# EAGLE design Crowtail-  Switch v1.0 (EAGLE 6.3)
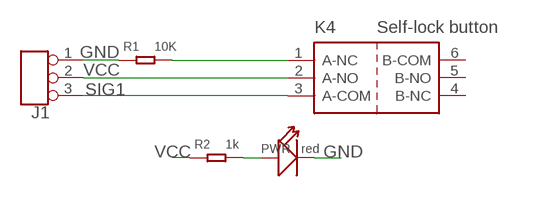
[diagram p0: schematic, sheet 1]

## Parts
J1  TINKER_3P_DIP  [3P_2.0_DIP]
K4  Self-lock button  BUTTON-6P  [6P-2CH-8X8]
PWR  red  LED'0603'  [LED-0603]
R1  10K  R-0603  [0603]
R2  1k  R-0603  [0603]

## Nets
GND: J1.1 PWR.- R1.1
N$1: PWR.+ R2.2
N$2: K4.1(A-NC) R1.2
SIG1: J1.3 K4.3(A-COM)
VCC: J1.2 K4.2(A-NO) R2.1
Unconnected: K4.4(B-NC) K4.5(B-NO) K4.6(B-COM)

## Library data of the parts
J1 = Connector:TINKER_3P_DIP
K4 = Discrete:BUTTON-6P
PWR = Discrete:LED*
R1 R2 = Discrete:R*

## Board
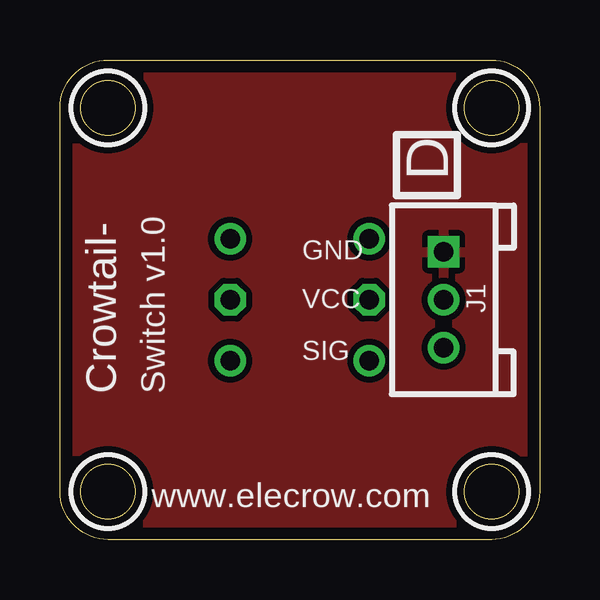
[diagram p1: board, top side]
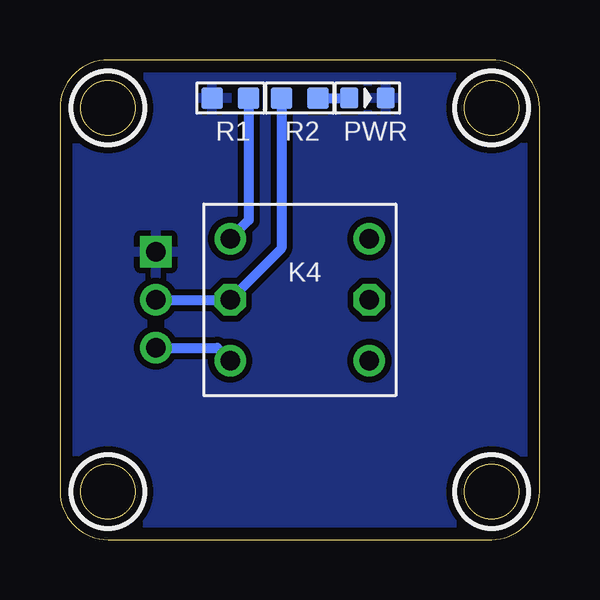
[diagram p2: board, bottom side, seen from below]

Size 20 x 20 mm. Coordinates in mm from the lower left corner, seen from the top.
Outline: 2,20 18,20 arc-90 20,18 20,2 arc-90 18,0 2,0 arc-90 0,2 0,18 arc-90 2,20
Outline: circle at 18,18 radius 1.14
Outline: circle at 18,2 radius 1.14
Outline: circle at 2,18 radius 1.14
Outline: circle at 2,2 radius 1.14
Copper layers (1*16): Top 0.035mm / dielectric 1.5mm / Bottom 0.035mm
Design rules "default": minimum track width 10mil, minimum drill 24mil, track to track 8mil, track to pad 8mil, pad to pad 8mil, via to via 8mil, smd to smd 8mil, copper to edge 20mil, drill to drill 8mil, minimum pad ring 10mil, minimum via ring 8mil, stop-mask expansion 4mil, vias tented up to drill 100mil, thermal gap 10mil
tRestrict: area 16.5,16.5 to 19.5,19.5; area 16.5,0.5 to 19.5,3.5; area 0.5,16.5 to 3.5,19.5; area 0.5,0.5 to 3.5,3.5
bRestrict: area 16.5,16.5 to 19.5,19.5; area 16.5,0.5 to 19.5,3.5; area 0.5,16.5 to 3.5,19.5; area 0.5,0.5 to 3.5,3.5

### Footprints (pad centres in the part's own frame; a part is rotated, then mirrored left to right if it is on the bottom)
3P_2.0_DIP = drill 0.8 pad 1.27 square: 1 -2,0 | drill 0.8 pad 1.27: 2 0,0; 3 2,0
6P-2CH-8X8 = drill 0.813 pad 1.27: 1 -2.9,2.54; 3 -2.9,-2.54; 4 2.9,-2.54; 6 2.9,2.54 | drill 0.813 pad 1.27 octagon: 2 -2.9,0; 5 2.9,0
LED-0603 = smd 0.762 x 0.889: + -0.762,0; - 0.762,0
0603 = smd 0.889 x 0.889: 1 -0.762,0; 2 0.762,0

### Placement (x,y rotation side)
J1  16,10 270 top
K4  10,10 0 bottom
PWR  7.17,18.41 0 bottom
R1  12.89,18.41 0 bottom
R2  10,18.41 0 bottom

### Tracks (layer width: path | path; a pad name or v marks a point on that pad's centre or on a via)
GND
  pour Top (isolate 0.254): 20,0 -0.32,0 -0.32,20.32 20,20.32
  pour Bottom (isolate 0.254): 20,0 -0.32,0 -0.32,20.19 20,20.19
N$1
  Bottom 0.406: R2.2 PWR.+
N$2
  Bottom 0.406: R1.2 12.13,13.31 K4.1
SIG1
  Bottom 0.406: J1.3 13.44,8 K4.3
VCC
  Bottom 0.406: J1.2 K4.2 10.76,12.14 R2.1

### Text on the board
tPlace: D | GND | VCC | SIG | Crowtail- | Switch v1.0 | www.elecrow.com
